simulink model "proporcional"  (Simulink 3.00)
settings: Solver=ode4  StartTime=0.0  StopTime=20  FixedStep=.0242  RelTol=1e-3
libraries: ballbeam x1

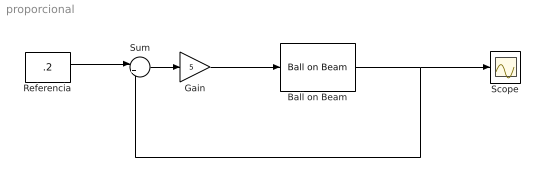
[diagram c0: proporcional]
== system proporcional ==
  Ball on Beam : ballbeam/Ball on Beam  v_ball=0  x_ball=.1
  Gain : Gain  Gain=5  SaturateOnIntegerOverflow=on
  Referencia : Constant  Value=.2
  Scope : Scope
  Sum : Sum  Inputs=|+-  SaturateOnIntegerOverflow=on
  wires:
  Referencia/1 -> Sum/1
  Sum/1 -> Gain/1
  Gain/1 -> Ball on Beam/1
  Ball on Beam/1 -> Scope/1, Sum/2
